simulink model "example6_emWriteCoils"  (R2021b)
settings: Solver=FixedStepAuto  StartTime=0  StopTime=inf  FixedStep=0.5  RelTol=1e-3  EnableMultiTasking=on
undefined symbols (not defined in the file or in its folder): based, classic, dsPic33, MCC, Microchip, PIC24
libraries: emMBSlaveLib x3, embeddedCreatorLib x1

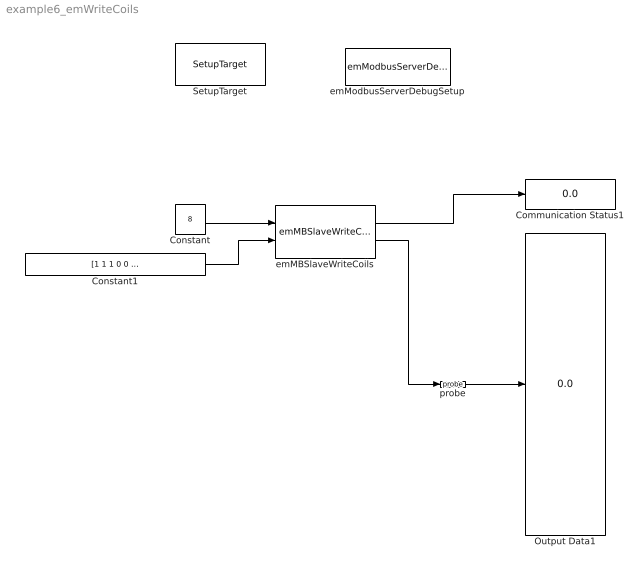
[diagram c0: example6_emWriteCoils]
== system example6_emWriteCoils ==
  Communication Status1 : Display
  Constant : Constant  Value=8  OutDataTypeStr=uint16
  Constant1 : Constant  Value=[1 1 1 0 0 0 1 1 1 0 0 0 1 1 1 1 1]  OutDataTypeStr=boolean
  Output Data1 : Display
  SetupTarget : embeddedCreatorLib/SetupTarget  Tag=SetupTarget  Priority=0  c_platform=Microchip PIC24/dsPic33 based on MCC classic  c_debug=on
  emMBSlaveWriteCoils : emMBSlaveLib/emMBSlaveWriteCoils  c_ServerID=1  c_UartNo=2  c_minAdr=8  c_RegQTY=18  c_singleWriting=off  c_sampleTime=-1
  emModbusServerDebugSetup : emMBSlaveLib/emModbusServerDebugSetup  Tag=emModbusSlaveSetup  c_objID=0  c_uartNo=2  c_baudrate=19200  c_serverID=1  c_baudrate4PC=19200  c_forceLongerSpace=on  c_holdingRegsQTY=0  c_minHoldingAddr=1  c_inputRegsQTY=0  c_minInputRegAddr=1  c_coilRegsQTY=18  c_minCoilAddr=8  c_discreteRegsQTY=0  c_minDiscreteAddr=8  c_enableDebug=on  c_breakpointMaxQTY=100  c_probeMaxWordQTY=200  c_emWaitQTY=0  g_COMPortNo=COM5  c_Name_method=By physical port name and bit number  c_PortName=B  c_BitNo=11  c_TxEnable485="\"LATBbits.LATB11\""  c_TxEnable485Polarity=on
  probe : emMBSlaveLib/probe  Tag=emProbe  c_ObjID=-1  c_serverID=1  c_UartNo=4  c_StartAddr=[]  c_ConstantDataSource=on
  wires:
  Constant/1 -> emMBSlaveWriteCoils/1
  emMBSlaveWriteCoils/1 -> Communication Status1/1
  Constant1/1 -> emMBSlaveWriteCoils/2
  emMBSlaveWriteCoils/2 -> probe/1
  probe/1 -> Output Data1/1
